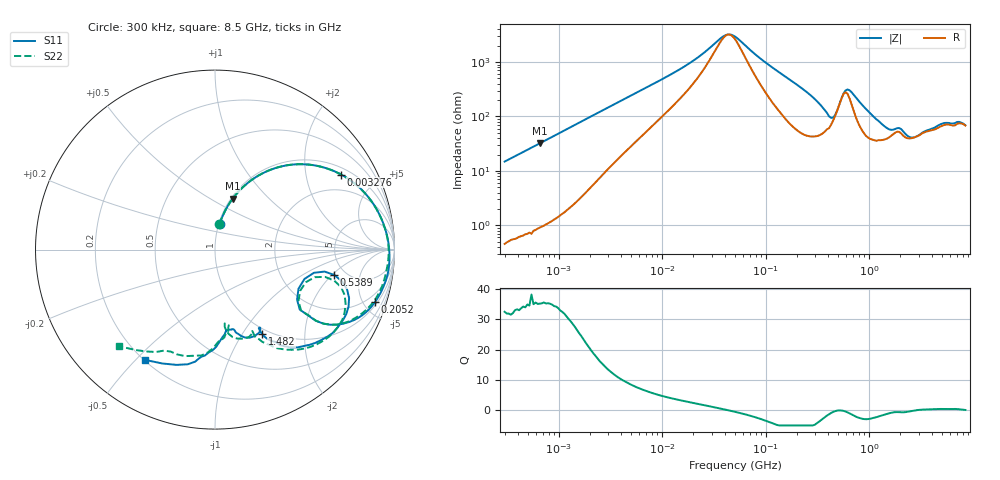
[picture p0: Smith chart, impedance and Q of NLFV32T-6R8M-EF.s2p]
! S-parameter Generated by TDK Corporation
! Copyright(C) 2015 TDK Corporation.
! All Rights Reserved.
! TDK P/N: NLFV32T-6R8M-EF (Inductors)
! Property: L=6.8uH at 7.96MHz
! Size(LxWxT): 3.2x2.5x2.2mm, 0.126x0.098x0.087inches
! Model Type: s2p (Touchstone File Format Version 1.0)
! Frequency: DC=Yes Start=0.3MHz Stop=8500MHz 225points Log-sweep
! Note:
! Model Generated on Jun. 23, 2015
! Hash(MD5):
! Port Assignments:
!  1 ---@@@--- 2
! Applicable Conditions:
!  Temperature = 25 degC
!  DC Bias Current = 0 A
!  Small Signal Operation
! Terms and conditions regarding TDK Simulation Models
! (1)This simulation model is being provided solely for informational purposes. Please refer to the specifications of the products in terms of detailed characteristics of such products.
! (2)In no event shall TDK Corporation of any of its subsidiaries be liable for any loss or damage arising, directly or indirectly,
!  From any information contained in this simulation model, including, but not limited to loss or damages arising from any inaccuracies, omissions or errors in connection with such information.
! (3)Any and all copyrights on this simulation model are owned by TDK Corporation.
!  Duplication or redistribution of this simulation model without prior written permission from TDK Corporation is prohibited.
! (4)This simulation model is subject to any modification or change without any prior notice.
! (5)Neither TDK Corporation nor any of its subsidiaries shall make any warranty, express or implied,
!  Including but not limited to the correctness, implied warranties of merchantability and fitness for a particular purpose with respect to this simulation models.
! (6)The use of this simulation model shall be deemed to have consented to the terms and conditions hereof.
# MHz S MA R 50
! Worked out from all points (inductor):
!   224 points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, 300 kHz to 8.5 GHz, reference 50 ohm
!   read as one part in series: L = 7.84 uH near 314.1 kHz
!   highest Q = 35.3 at 655.4 kHz (marker M1), where L = 7.78 uH
!   self-resonance near 43.68 MHz
!   S11 on the Smith chart (normalised r, x): 300 kHz: 1.01, +0.29; 3.276 MHz: 1.26, +3.19; 205.2 MHz: 1.23, -5.98; 538.9 MHz: 4.06, -2.13; 1.482 GHz: 0.93, -1.23; 8.5 GHz: 0.20, -0.53
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0.3  0.1445 79.9  0.9828 -8.4  0.9874 -8.6  0.1437 80.1
0.6554417  0.3011 70.8  0.9449 -17.6  0.9468 -17.9  0.3009 70.8
1.72111  0.6302 48.5  0.7509 -39.1  0.7521 -39.4  0.6307 48.5
3.275859  0.8184 30.7  0.5138 -54.7  0.5145 -55.1  0.819 30.6
9.430415  0.9393 11.4  0.2058 -67.3  0.2059 -67.6  0.9395 11.3
20.60362  0.9629 4.2  0.08725 -62.7  0.0873 -63.0  0.9622 4.0
39.21571  0.9708 -0.2  0.03246 -19.6  0.03249 -20.0  0.9678 -0.4
51.67171  0.9727 -2.0  0.034 27.8  0.03402 27.5  0.9677 -2.2
205.2186  0.9377 -18.2  0.2486 63.2  0.2487 62.9  0.9268 -18.7
283.1228  0.8688 -26.8  0.3685 52.4  0.3687 52.1  0.8578 -27.1
356.2888  0.7292 -34.4  0.481 36.8  0.4812 36.4  0.731 -34.3
428.2171  0.5356 -31.4  0.5388 13.6  0.5395 13.1  0.5469 -31.7
538.8791  0.6794 -12.0  0.3173 -7.2  0.3173 -7.6  0.6865 -14.6
618.5683  0.7943 -19.8  0.2441 14.7  0.2442 14.4  0.7881 -22.6
893.5346  0.7632 -42.9  0.4522 28.7  0.4532 28.1  0.7601 -45.4
1481.602  0.5372 -60.8  0.6133 -1.0  0.6138 -1.6  0.5387 -65.2
1551.304  0.5184 -61.0  0.6142 -4.0  0.6144 -4.8  0.5201 -65.4
2572.272  0.4783 -75.7  0.6195 -27.9  0.6196 -28.6  0.447 -82.4
4073.536  0.4547 -81.9  0.5202 -57.6  0.5231 -58.7  0.5019 -85.6
5126.239  0.5183 -87.6  0.4337 -73.1  0.4328 -73.5  0.5747 -94.0
7072.242  0.6344 -100.1  0.314 -92.8  0.3153 -93.6  0.6587 -120.0
8500  0.7277 -122.4  0.2268 -96.1  0.2262 -95.3  0.7609 -134.9
